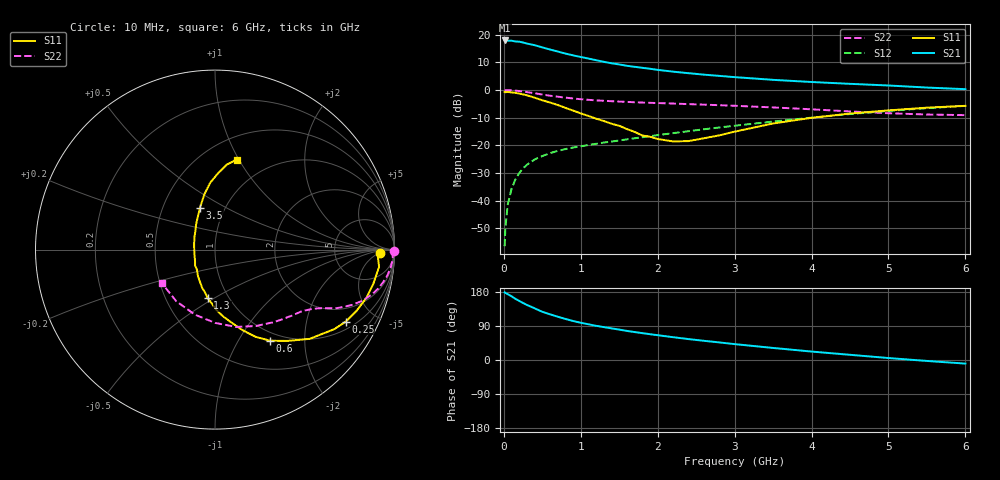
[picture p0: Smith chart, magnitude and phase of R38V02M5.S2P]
! SIEMENS Small Signal Semiconductors
! BFR181
! Si NPN RF Bipolar Junction Transistor in SOT23
! VCE = 8 V  IC = 2.5 mA
! Common Emitter S-Parameters:  May  1996
# GHz  S  MA  R  50
!  f  S11  S21  S12  S22
! GHz  MAG  ANG  MAG  ANG  MAG  ANG  MAG  ANG
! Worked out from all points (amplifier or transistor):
!   36 points, 10 MHz to 6 GHz, reference 50 ohm
!   highest |S21| = 17.9 dB at 10 MHz (marker M1)
!   |S21| within 3 dB of that: start of sweep to 564.5 MHz
!   unconditionally stable (mu >= 1): 1.535 GHz to 3.375 GHz
!   at 250 MHz: K = 0.26, MSG = 22.8 dB, |S12| = -28.4 dB
!   at 1.4 GHz: K = 0.97, MSG = 14.2 dB, |S12| = -18.7 dB
!   at 6 GHz: K = 0.86, MSG = 3.0 dB, |S12| = -5.8 dB
!   S11 on the Smith chart (normalised r, x): 10 MHz: 22, -5; 250 MHz: 1.31, -3.41; 600 MHz: 0.88, -1.37; 1.3 GHz: 0.80, -0.47; 3.5 GHz: 0.76, +0.38; 6 GHz: 0.72, +0.98
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0.01  0.9188 -1.1  7.838 178.5  0.0015 88.7  0.996 -0.5
0.02  0.9082 -2.4  7.605 177.1  0.0032 85.8  0.9902 -1.2
0.05  0.9191 -6.0  7.785 173.8  0.0084 84.6  0.9919 -2.9
0.1  0.9027 -12.1  7.747 168.1  0.0163 83.0  0.9842 -5.7
0.15  0.8861 -17.5  7.514 161.4  0.0241 79.6  0.9715 -8.5
0.2  0.8593 -23.4  7.441 155.9  0.0314 76.7  0.954 -11.0
0.25  0.8312 -28.9  7.199 150.4  0.0382 73.4  0.9352 -13.4
0.3  0.7987 -33.7  6.881 145.3  0.0444 71.1  0.9139 -15.5
0.4  0.7251 -43.3  6.438 136.4  0.0554 66.9  0.8713 -19.0
0.5  0.6493 -51.6  5.876 127.2  0.0637 63.3  0.8249 -21.9
0.6  0.5927 -58.9  5.377 120.6  0.0721 61.0  0.786 -23.9
0.8  0.4744 -71.1  4.542 108.4  0.0852 57.5  0.7269 -26.7
0.9  0.4231 -76.5  4.217 102.9  0.0909 56.9  0.7004 -27.8
1.1  0.3392 -88.3  3.689 94.3  0.1011 56.6  0.6625 -29.6
1.3  0.2745 -98.5  3.221 86.8  0.1119 56.4  0.6357 -31.3
1.7  0.1744 -123.1  2.617 73.7  0.1337 57.1  0.5987 -34.7
2.2  0.1173 -168.1  2.139 60.2  0.1655 57.5  0.5678 -40.2
2.6  0.1337 149.2  1.889 50.7  0.1944 56.9  0.5422 -45.5
3.5  0.2477 109.8  1.521 31.8  0.2682 53.1  0.4831 -61.8
4.5  0.3744 94.0  1.289 13.7  0.3664 44.6  0.4084 -89.9
5.5  0.478 82.1  1.104 -2.5  0.4677 32.6  0.3595 -127.0
6  0.516 76.5  1.032 -9.5  0.5148 25.6  0.3502 -147.5
